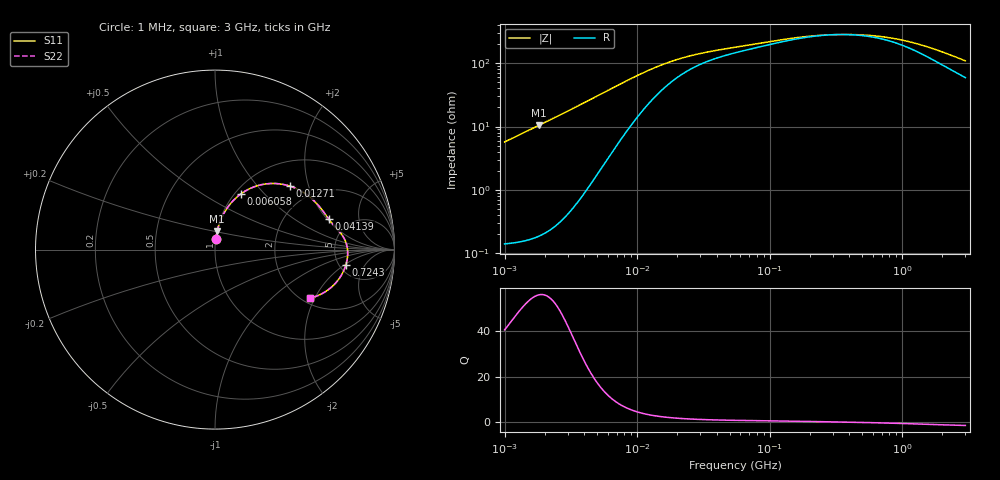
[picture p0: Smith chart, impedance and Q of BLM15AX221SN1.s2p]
! BLM15AX221SN1
# Hz S RI R 50
!Freq.(Hz) S11(Real) S11(Imag) S21(Real) S21(Imag) S12(Real) S12(Imag) S22(Real) S22(Imag)
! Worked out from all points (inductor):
!   401 points, 1 MHz to 3 GHz, reference 50 ohm
!   read as one part in series: L = 911 nH near 1.041 MHz
!   highest Q = 56.1 at 1.823 MHz (marker M1), where L = 916 nH
!   self-resonance near 321.7 MHz
!   S11 on the Smith chart (normalised r, x): 1 MHz: 1.00, +0.11; 6.058 MHz: 1.06, +0.74; 12.71 MHz: 1.50, +1.52; 41.39 MHz: 3.46, +2.09; 724.3 MHz: 5.75, -2.10; 3 GHz: 2.18, -1.82
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1000000  0.00464 0.0567  0.9954 -0.0567  0.9954 -0.0567  0.00464 0.0567
1822989  0.0127 0.1033  0.9873 -0.1033  0.9873 -0.1033  0.0127 0.1033
2666535  0.0265 0.1506  0.9735 -0.1506  0.9735 -0.1506  0.0265 0.1506
3823119  0.0556 0.2126  0.9444 -0.2126  0.9444 -0.2126  0.0556 0.2126
4861065  0.0916 0.2624  0.9084 -0.2624  0.9084 -0.2624  0.0916 0.2624
6058321  0.1425 0.3092  0.8575 -0.3092  0.8575 -0.3092  0.1425 0.3092
8861669  0.2741 0.3645  0.7259 -0.3645  0.7259 -0.3645  0.2741 0.3645
1.061086e7  0.3468 0.3676  0.6532 -0.3676  0.6532 -0.3676  0.3468 0.3676
1.270533e7  0.4158 0.3542  0.5842 -0.3542  0.5842 -0.3542  0.4158 0.3542
1.461624e7  0.463 0.3352  0.537 -0.3352  0.537 -0.3352  0.463 0.3352
1.821614e7  0.5228 0.2972  0.4772 -0.2972  0.4772 -0.2972  0.5228 0.2972
2.270269e7  0.5659 0.2574  0.4341 -0.2574  0.4341 -0.2574  0.5659 0.2574
4.138676e7  0.6326 0.1722  0.3674 -0.1722  0.3674 -0.1722  0.6326 0.1722
5.477226e7  0.6534 0.1454  0.3466 -0.1454  0.3466 -0.1454  0.6534 0.1454
2.094008e8  0.7301 0.038  0.2699 -0.038  0.2699 -0.038  0.7301 0.038
3.973271e8  0.7394 -0.0197  0.2606 0.0197  0.2606 0.0197  0.7394 -0.0197
7.243229e8  0.7297 -0.0841  0.2703 0.0841  0.2703 0.0841  0.7297 -0.0841
8.005644e8  0.7257 -0.0965  0.2743 0.0965  0.2743 0.0965  0.7257 -0.0965
1.10276e9  0.7055 -0.1403  0.2945 0.1403  0.2945 0.1403  0.7055 -0.1403
1.581072e9  0.6643 -0.1946  0.3357 0.1946  0.3357 0.1946  0.6643 -0.1946
2.092429e9  0.6143 -0.235  0.3857 0.235  0.3857 0.235  0.6143 -0.235
3e9  0.5266 -0.2711  0.4734 0.2711  0.4734 0.2711  0.5266 -0.2711
